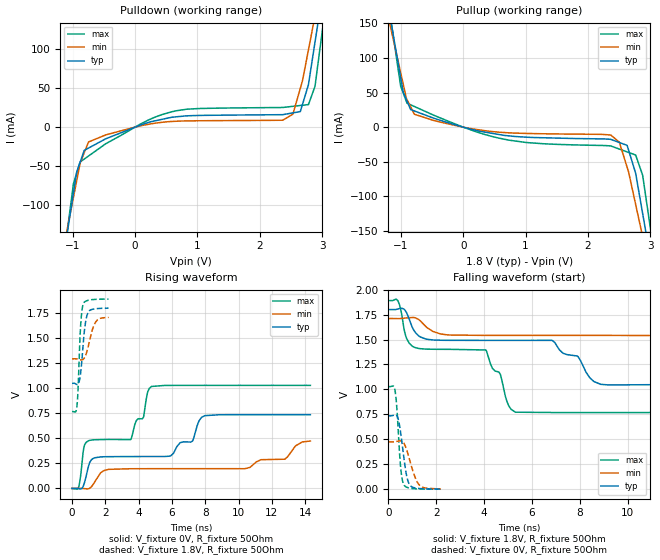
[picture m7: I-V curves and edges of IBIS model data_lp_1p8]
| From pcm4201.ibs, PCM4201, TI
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|   data_lp_1p8 Model
[Model]   data_lp_1p8
Model_type   Output
Polarity   Non-Inverting
Vmeas = 0.9
Vref = 0.9
Cref = 2pF
Rref = 50
|   typ   min   max
|   (nom PVT)   (fast PVT)   (slow PVT)
|C_comp from frequency sweep method (F=13.83MHz)
|C_comp   1.509e-12   1.305e-12   1.737e-12
|ON state : BUFFER OUTPUT TURNED HIGH
|C_comp   1.509e-12   1.305e-12   1.737e-12
|OFF state: BUFFER OUTPUT TURNED LOW
|C_comp   1.516e-12   1.344e-12   1.678e-12
|C_comp from LC tank measurement(L=1nH)
|Resonant Frequency(Hz)   7.400e+09   7.640e+09   7.170e+09
C_comp   4.630e-13   4.344e-13   4.932e-13
|ON state : BUFFER OUTPUT TURNED HIGH
|Resonant Frequency(Hz)   7.400e+09   7.640e+09   7.170e+09
|C_comp   4.630e-13   4.344e-13   4.932e-13
|OFF state: BUFFER OUTPUT TURNED LOW
|Resonant Frequency(Hz)   7.400e+09   7.680e+09   7.150e+09
|C_comp   4.630e-13   4.299e-13   4.960e-13
| Where nom  PVT is Nominal Process, 1.8V, 35C
|   Fast PVT is Strong Process,  1.89V, -10C
|   Slow PVT is Weak Process,   1.71V, 80C
[Voltage Range]   1.8   1.71   1.89
|Ambient Temperature   25   70   -10
|Junction Temperature
[Temperature Range]   35   80   -10
[Pullup Reference]   1.8   1.71   1.89
[Pulldown Reference]   0   0   0
[Power Clamp Reference]   1.8   1.71   1.89
[GND Clamp Reference]   0   0   0
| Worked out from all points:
|   slope of the pulldown table from 0 to 0.27 V, typ, clamps not added: 37.4 ohm
|   slope of the pullup table from 0 to 0.27 V, typ, clamps not added: 45.3 ohm
|   falling waveform, V_fixture 1.8V, R_fixture 50Ohm: 20-80 % time 7.25ns typ, 12.9ns min, 4.22ns max; typ from 1.8 V to 1.05 V
|   rising waveform, V_fixture 0V, R_fixture 50Ohm: 20-80 % time 6.57ns typ, 11.7ns min, 3.83ns max; typ from 0 V to 0.736 V
|   rising waveform, V_fixture 1.8V, R_fixture 50Ohm: 20-80 % time 256ps typ, 400ps min, 171ps max; typ from 1.05 V to 1.8 V
|   falling waveform, V_fixture 0V, R_fixture 50Ohm: 20-80 % time 252ps typ, 372ps min, 167ps max; typ from 0.736 V to 0.002 V
[Pulldown]
|   Voltage   I(typ)   I(min)   I(max)
-1.8V     -507.1mA   -421.2mA   -630.4mA
-1.238V   -213.8mA   -192.2mA   -227.7mA
-988.5mV  -85.08mA   -90.63mA   -73.25mA
-813.6mV  -29.73mA   -32.72mA   -40.9mA
-471.6mV  -15.02mA   -10.01mA   -21.4mA
653.9mV   13.19mA    7.521mA    20.87mA
2.365V    15.98mA    8.874mA    25.2mA
2.529V    18.28mA    16.57mA    26.68mA
2.648V    19.95mA    49.71mA    27.75mA
2.884V    109.4mA    143.1mA    52.93mA
3.103V    222.9mA    234.2mA    186mA
3.6V      486.1mA    440.5mA    540.3mA
[Pullup]
|   Voltage   I(typ)   I(min)   I(max)
-1.8V     486.4mA    402.6mA    606.4mA
-1.246V   197.3mA    177.6mA    208.7mA
-1.002V   71.71mA    78.73mA    59.22mA
-783.2mV  23.41mA    18.65mA    29.85mA
655.8mV   -11.9mA    -7.77mA    -17.45mA
2.365V    -17.68mA   -11.38mA   -27.18mA
2.502V    -22.19mA   -21.76mA   -31.68mA
2.626V    -26.29mA   -57.91mA   -35.78mA
2.763V    -66.63mA   -111.7mA   -40.28mA
2.875V    -124.5mA   -158mA     -69.36mA
3.103V    -243.3mA   -252.9mA   -210.3mA
3.6V      -506.9mA   -458.9mA   -564.5mA
[Ramp]
R_load = 50
|   typ   min   max
dV/dt_r   0.441654/6.56557e-09   0.284902/1.17403e-08   0.617078/3.82869e-09
dV/dt_f   0.450589/7.24618e-09   0.250182/1.29318e-08   0.672895/4.2138e-09
[Falling Waveform]
V_fixture = 1.8V
V_fixture_min = 1.71V
V_fixture_max = 1.89V
R_fixture = 50Ohm
|   Time   V(typ)   V(min)   V(max)
0s        1.8V       1.71V      1.89V
400ps     1.805V     1.71V      1.889V
736ps     1.78V      1.716V     1.529V
1.064ns   1.593V     1.72V      1.425V
4.072ns   1.491V     1.541V     1.395V
5.312ns   1.491V     1.541V     772mV
6.856ns   1.489V     1.541V     768.8mV
8.872ns   1.051V     1.541V     768.5mV
12.11ns   1.049V     1.538V     768.5mV
15.99ns   1.049V     1.293V     768.5mV
[Rising Waveform]
V_fixture = 0V
V_fixture_min = 0V
V_fixture_max = 0V
R_fixture = 50Ohm
|   Time   V(typ)   V(min)   V(max)
0s        642.3pV    1.279nV    373.2pV
392ps     -2.051mV   310uV      12.04mV
816ps     102.4mV    -3.413mV   453.2mV
1.304ns   302mV      49.97mV    484.8mV
3.52ns    318.2mV    196.4mV    487.5mV
4.776ns   318.4mV    196.8mV    1.017V
7.232ns   473.3mV    197mV      1.028V
7.96ns    725.8mV    197mV      1.028V
12.78ns   736.1mV    291.6mV    1.028V
14.31ns   736.1mV    473.3mV    1.028V
[Rising Waveform]
V_fixture = 1.8V
V_fixture_min = 1.71V
V_fixture_max = 1.89V
R_fixture = 50Ohm
|   Time   V(typ)   V(min)   V(max)
0s        1.049V     1.293V     768.5mV
208ps     1.044V     1.293V     763.3mV
296ps     1.037V     1.292V     826.6mV
360ps     1.04V      1.289V     993.3mV
512ps     1.15V      1.283V     1.618V
664ps     1.432V     1.287V     1.838V
808ps     1.657V     1.326V     1.867V
976ps     1.762V     1.419V     1.877V
1.416ns   1.793V     1.659V     1.886V
2.192ns   1.799V     1.707V     1.889V
[Falling Waveform]
V_fixture = 0V
V_fixture_min = 0V
V_fixture_max = 0V
R_fixture = 50Ohm
|   Time   V(typ)   V(min)   V(max)
0s        736.1mV    475.1mV    1.028V
208ps     739.8mV    474.8mV    1.034V
288ps     745.6mV    476.7mV    979.5mV
360ps     736.9mV    479.6mV    803.9mV
512ps     573.9mV    484.9mV    230.7mV
640ps     335.4mV    464.3mV    49.94mV
776ps     124.3mV    388.1mV    20.02mV
928ps     32.96mV    261.9mV    9.632mV
1.36ns    6.082mV    27.76mV    3.215mV
2.192ns   1.68mV     2.824mV    1.013mV
